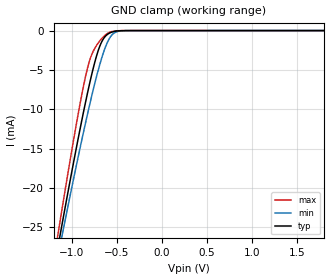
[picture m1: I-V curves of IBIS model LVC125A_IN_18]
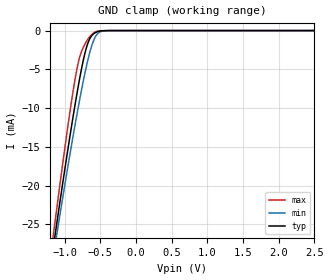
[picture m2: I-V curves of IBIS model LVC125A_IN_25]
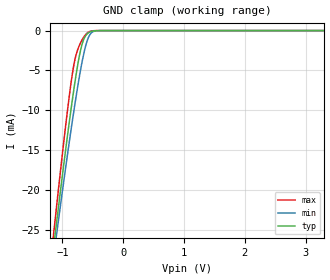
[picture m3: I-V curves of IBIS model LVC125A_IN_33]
| TEXAS INSTRUMENTS INCORPORATED
| Standard Linear and Logic Group
| IBIS Model of SN74LVC125A
| QUADRUPLE BUS BUFFER GATE WITH 3-STATE OUTPUTS
| This file contains package information for the following:
|  SOIC 14-pin (D) package as [Component] LVC125A_D
|  SSOP 14-pin (DB) package as [Component] LVC125A_DB
|  SOP 14-pin (NS) package as [Component] LVC125A_NS
|  TSSOP 14-pin (PW) package as [Component] LVC125A_PW
|  QFN 14-pin (RGY) package as [Component] LVC125A_RGY
| This device can be powered at the following Vccs:
|  1.8 volt Vcc
|  2.5 volt Vcc
|  3.3 volt Vcc
| This file provides unique models under the [Model Selector] for each Vcc.
| For operation at a specific Vcc, select the appropriate model after each
| [Model Selector] keyword.
[IBIS Ver]   4.1
[File Name]   sn74lvc125a.ibs
[File Rev]   1.2
[Date]   February 18, 2016
[Source]   Data created from TI-SPICE simulations at:
   Texas Instruments Incorporated.
   Analog-eLab, HPA
   12500 TI Blvd
   Dallas, TX -75243
   For Support e-mail: elab_ibis@list.ti.com
[Notes]   The following is an IBIS list for the LVC125A.
   Please contact sllibis@ti.com with questions and
   comments concerning SLL IBIS models.
   Rev 1.2: 2/18/16
   - Add RGY package component
   Rev 1.1: 5/23/02
   - Model avaiable on product folder
[Disclaimer]  This model is designed as an aid for customers of Texas Instruments
 TI and its licensors and suppliers make no warranties, either expressed
 or implied, with respect to this  model, including the warranties of
 merchantability or fitness for a particular purpose.
 The model is provided solely on an "as is" basis. The entire risk as to
 its quality and performance is with the customer.
[Copyright] (C)Copyright 2016 Texas Instruments Incorporated.
   All rights reserved.
| Component LVC125A_D 14-pin SOIC
[Component]   LVC125A_D
[Manufacturer]   Texas Instruments, Inc.
[Package]
|   typ   min   max
R_pkg   3.100e-02   2.800e-02   3.400e-02
L_pkg   3.109e-09   2.462e-09   3.889e-09
C_pkg   4.730e-13   3.630e-13   6.280e-13
[Pin]   signal_name   model_name   R_pin   L_pin   C_pin
1   1NOE   LVC125A_IN   3.300e-02   3.854e-09   6.220e-13
2   1A   LVC125A_IN   3.200e-02   3.188e-09   4.730e-13
3   1Y   LVC125A_OUT   2.800e-02   2.462e-09   3.770e-13
4   2NOE   LVC125A_IN   3.100e-02   2.596e-09   3.630e-13
5   2A   LVC125A_IN   2.800e-02   2.521e-09   3.720e-13
6   2Y   LVC125A_OUT   3.400e-02   3.250e-09   4.760e-13
7   GND   GND   3.400e-02   3.889e-09   6.280e-13
8   3Y   LVC125A_OUT   3.400e-02   3.889e-09   6.280e-13
9   3A   LVC125A_IN   3.400e-02   3.250e-09   4.760e-13
10   3NOE   LVC125A_IN   2.800e-02   2.521e-09   3.720e-13
11   4Y   LVC125A_OUT   3.100e-02   2.596e-09   3.640e-13
12   4A   LVC125A_IN   2.800e-02   2.462e-09   3.770e-13
13   4NOE   LVC125A_IN   3.200e-02   3.188e-09   4.730e-13
14   VCC   POWER   3.300e-02   3.854e-09   6.220e-13
| Component LVC125A_DB 14-pin SSOP
[Component]   LVC125A_DB
[Manufacturer]   Texas Instruments, Inc.
[Package]
|   typ   min   max
R_pkg   4.400e-02   4.100e-02   4.600e-02
L_pkg   3.551e-09   3.258e-09   3.927e-09
C_pkg   4.020e-13   3.600e-13   4.210e-13
[Pin]   signal_name   model_name   R_pin   L_pin   C_pin
1   1NOE   LVC125A_IN   4.600e-02   3.927e-09   4.080e-13
2   1A   LVC125A_IN   4.400e-02   3.587e-09   4.210e-13
3   1Y   LVC125A_OUT   4.100e-02   3.289e-09   3.980e-13
4   2NOE   LVC125A_IN   4.200e-02   3.258e-09   3.600e-13
5   2A   LVC125A_IN   4.100e-02   3.286e-09   4.030e-13
6   2Y   LVC125A_OUT   4.400e-02   3.586e-09   4.210e-13
7   GND   GND   4.600e-02   3.927e-09   4.080e-13
8   3Y   LVC125A_OUT   4.600e-02   3.927e-09   4.080e-13
9   3A   LVC125A_IN   4.400e-02   3.586e-09   4.210e-13
10   3NOE   LVC125A_IN   4.100e-02   3.286e-09   4.030e-13
11   4Y   LVC125A_OUT   4.300e-02   3.258e-09   3.600e-13
12   4A   LVC125A_IN   4.100e-02   3.289e-09   3.980e-13
13   4NOE   LVC125A_IN   4.400e-02   3.587e-09   4.210e-13
14   VCC   POWER   4.600e-02   3.927e-09   4.080e-13
| Component LVC125A_NS 14-pin SOP
[Component]   LVC125A_NS
[Manufacturer]   Texas Instruments, Inc.
[Package]
|   typ   min   max
R_pkg   4.500e-02   3.900e-02   5.400e-02
L_pkg   3.796e-09   2.561e-09   4.952e-09
C_pkg   5.280e-13   2.880e-13   7.100e-13
[Pin]   signal_name   model_name   R_pin   L_pin   C_pin
1   1NOE   LVC125A_IN   4.700e-02   4.867e-09   7.060e-13
2   1A   LVC125A_IN   5.100e-02   4.083e-09   5.920e-13
3   1Y   LVC125A_OUT   4.100e-02   2.915e-09   3.760e-13
4   2NOE   LVC125A_IN   3.900e-02   2.561e-09   2.880e-13
5   2A   LVC125A_IN   4.100e-02   3.101e-09   4.300e-13
6   2Y   LVC125A_OUT   4.700e-02   4.047e-09   5.890e-13
7   GND   GND   5.100e-02   4.909e-09   7.000e-13
8   3Y   LVC125A_OUT   4.500e-02   4.784e-09   6.940e-13
9   3A   LVC125A_IN   5.400e-02   4.176e-09   5.970e-13
10   3NOE   LVC125A_IN   3.900e-02   3.287e-09   4.490e-13
11   4Y   LVC125A_OUT   3.900e-02   2.586e-09   2.940e-13
12   4A   LVC125A_IN   4.000e-02   2.802e-09   3.710e-13
13   4NOE   LVC125A_IN   4.900e-02   4.080e-09   5.930e-13
14   VCC   POWER   5.200e-02   4.952e-09   7.100e-13
| Component LVC125A_PW 14-pin TSSOP
[Component]   LVC125A_PW
[Manufacturer]   Texas Instruments, Inc.
[Package]
|   typ   min   max
R_pkg   3.200e-02   2.900e-02   3.500e-02
L_pkg   2.378e-09   2.170e-09   2.680e-09
C_pkg   3.140e-13   2.700e-13   3.350e-13
[Pin]   signal_name   model_name   R_pin   L_pin   C_pin
1   1NOE   LVC125A_IN   3.300e-02   2.618e-09   3.300e-13
2   1A   LVC125A_IN   3.100e-02   2.313e-09   3.170e-13
3   1Y   LVC125A_OUT   3.000e-02   2.310e-09   3.140e-13
4   2NOE   LVC125A_IN   3.100e-02   2.173e-09   2.720e-13
5   2A   LVC125A_IN   3.000e-02   2.204e-09   3.090e-13
6   2Y   LVC125A_OUT   3.200e-02   2.315e-09   3.170e-13
7   GND   GND   3.500e-02   2.680e-09   3.350e-13
8   3Y   LVC125A_OUT   3.300e-02   2.640e-09   3.330e-13
9   3A   LVC125A_IN   3.400e-02   2.347e-09   3.190e-13
10   3NOE   LVC125A_IN   2.900e-02   2.277e-09   3.130e-13
11   4Y   LVC125A_OUT   3.100e-02   2.170e-09   2.700e-13
12   4A   LVC125A_IN   3.100e-02   2.244e-09   3.110e-13
13   4NOE   LVC125A_IN   3.300e-02   2.343e-09   3.210e-13
14   VCC   POWER   3.500e-02   2.657e-09   3.320e-13
| Component LVC125A_RGY 14-pin QFN
[Component]   LVC125A_RGY
[Manufacturer]   Texas Instruments, Inc.
[Package]   |14-pin QFN (RGY)
|   typ   min   max
R_pkg   0.099   0.110   0.089
L_pkg   1.340n   1.497n   1.198n
C_pkg   0.134p   0.144p   0.112p
[Pin]   signal_name   model_name   R_pin   L_pin   C_pin
1   1NOE   LVC125A_IN   0.10053   1.37155n   0.12253p
2   1A   LVC125A_IN   0.10362   1.41529n   0.13900p
3   1Y   LVC125A_OUT   0.08967   1.20546n   0.13617p
4   2NOE   LVC125A_IN   0.08916   1.19759n   0.13490p
5   2A   LVC125A_IN   0.09214   1.24186n   0.13836p
6   2Y   LVC125A_OUT   0.10306   1.40689n   0.13750p
7   GND   GND   0.10160   1.38688n   0.12415p
8   3Y   LVC125A_OUT   0.10659   1.45718n   0.12766p
9   3A   LVC125A_IN   0.10966   1.49669n   0.14417p
10   3NOE   LVC125A_IN   0.09474   1.27156n   0.14062p
11   4Y   LVC125A_OUT   0.09359   1.25409n   0.13866p
12   4A   LVC125A_IN   0.09527   1.27936n   0.14089p
13   4NOE   LVC125A_IN   0.10515   1.42940n   0.13914p
14   VCC   POWER   0.09951   1.34780n   0.11157p
| Model LVC125A_IN
[Model Selector]   LVC125A_IN
LVC125A_IN_18   1.8 volt Vcc
LVC125A_IN_25   2.5 volt Vcc
LVC125A_IN_33   3.3 volt Vcc
| Model LVC125A_OUT
[Model Selector]   LVC125A_OUT
LVC125A_OUT_18   1.8 volt Vcc
LVC125A_OUT_25   2.5 volt Vcc
LVC125A_OUT_33   3.3 volt Vcc
| Models and submodels in the file (6): LVC125A_IN_18 (Input), LVC125A_IN_25 (Input), LVC125A_IN_33 (Input), LVC125A_OUT_18 (3-state), LVC125A_OUT_25 (3-state), LVC125A_OUT_33 (3-state)
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[Model]   LVC125A_IN_18
Model_type  Input
Vinl=0.5775
Vinh=1.2675
| variable   typ   min   max
C_comp   2.66pF   2.19pF   3.17pF
[Temperature Range]   40   100   -40
| Ambient temperature   25   85   -40
[Voltage range]   1.8   1.65   1.95
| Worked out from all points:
|   GND clamp passes 1 mA (typ) near -0.64 V on its own axis
[GND Clamp]
| LVC125A_IN_18
|   Voltage   I(typ)   I(min)   I(max)
-5.5V     -338.9mA   -314.3mA   -369mA
-1.16V    -28.09mA   -29.24mA   -26.56mA
-1.12V    -25.56mA   -26.92mA   -23.71mA
-1.085V   -23.36mA   -24.91mA   -21.25mA
-925mV    -13.65mA   -15.98mA   -10.52mA
-820mV    -7.797mA   -10.48mA   -4.654mA
-770mV    -5.293mA   -8.026mA   -2.891mA
-695mV    -2.253mA   -4.666mA   -1.432mA
-600mV    -473.7uA   -1.449mA   -358.4uA
-535mV    -136.2uA   -379.8uA   -78.5uA
-445mV    -16.2uA    -36.49uA   -4.833uA
1.8V      41.95pA    147.4pA    23.47pA
[Model]   LVC125A_IN_25
Model_type  Input
Vinl=0.7
Vinh=1.7
| variable   typ   min   max
C_comp   2.58pF   2.03pF   3.24pF
[Temperature Range]   40   100   -40
| Ambient temperature   25   85   -40
[Voltage range]   2.5   2.3   2.7
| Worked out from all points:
|   GND clamp passes 1 mA (typ) near -0.64 V on its own axis
[GND Clamp]
| LVC125A_IN_25
|   Voltage   I(typ)   I(min)   I(max)
-5.5V     -338.9mA   -314.3mA   -369mA
-1.17V    -28.73mA   -29.82mA   -27.27mA
-1.13V    -26.19mA   -27.5mA    -24.42mA
-1.095V   -23.98mA   -25.48mA   -21.95mA
-925mV    -13.65mA   -15.98mA   -10.52mA
-825mV    -8.06mA    -10.74mA   -4.88mA
-775mV    -5.531mA   -8.266mA   -3.027mA
-700mV    -2.416mA   -4.874mA   -1.51mA
-590mV    -396.4uA   -1.217mA   -293.2uA
-515mV    -88.16uA   -231.8uA   -44.89uA
-395mV    -4.232uA   -9.445uA   -775nA
2.5V      57.25pA    176.8pA    32.61pA
[Model]   LVC125A_IN_33
Model_type  Input
Vinl=0.8
Vinh=2.0
| variable   typ   min   max
C_comp   2.50pF   1.92pF   3.16pF
[Temperature Range]   40   100   -40
| Ambient temperature   25   85   -40
[Voltage range]   3.3   3   3.6
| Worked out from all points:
|   GND clamp passes 1 mA (typ) near -0.64 V on its own axis
[GND Clamp]
| LVC125A_IN_33
|   Voltage   I(typ)   I(min)   I(max)
-5.5V     -338.9mA   -314.3mA   -369mA
-1.14V    -26.82mA   -28.07mA   -25.13mA
-1.105V   -24.61mA   -26.05mA   -22.65mA
-1.075V   -22.73mA   -24.34mA   -20.55mA
-915mV    -13.07mA   -15.45mA   -9.893mA
-860mV    -9.954mA   -12.53mA   -6.658mA
-805mV    -7.019mA   -9.733mA   -4.027mA
-730mV    -3.528mA   -6.174mA   -2.02mA
-665mV    -1.428mA   -3.486mA   -1.009mA
-585mV    -362.1uA   -1.111mA   -263.9uA
-510mV    -78.77uA   -204.1uA   -38.82uA
3.3V      76.2pA     212.8pA    43.07pA
